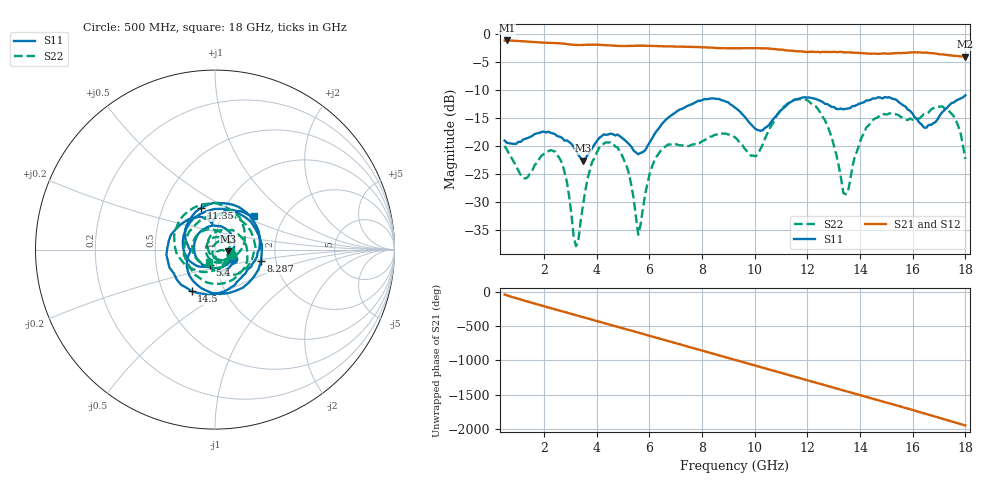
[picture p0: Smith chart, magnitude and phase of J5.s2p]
!Agilent Technologies,N5230A,MY45001360,A.07.50.67
!Agilent N5230A: A.07.50.67
!Date: Tuesday, April 16, 2024 15:56:14
!Correction: S11(Full 2 Port(1,2))
!S21(Full 2 Port(1,2))
!S12(Full 2 Port(1,2))
!S22(Full 2 Port(1,2))
!S2P File: Measurements: S11, S21, S12, S22:
# Hz S  dB  R 50
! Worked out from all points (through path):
!   201 points, 500 MHz to 18 GHz, reference 50 ohm
!   highest |S21| = -1.19 dB at 587.5 MHz (marker M1); lowest = -4.1 dB at 18 GHz (marker M2)
!   group delay of S21, straight-line fit = 300 ps
!   lowest |S11| = -22.6 dB at 3.475 GHz (marker M3), VSWR 1.16, Z = 57.9 - j1.15 ohm
!   |S11| at or under -10 dB: start of sweep to end of sweep
!   |S22| runs from -37.8 to -11.6 dB; largest |S21 - S12| = 0.0072
!   S11 on the Smith chart (normalised r, x): 500 MHz: 1.21, -0.13; 5.4 GHz: 0.93, -0.16; 8.287 GHz: 1.67, -0.23; 11.35 GHz: 0.77, +0.38; 14.5 GHz: 0.70, -0.35; 18 GHz: 1.41, +0.57
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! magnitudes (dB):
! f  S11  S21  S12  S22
! 500 MHz  -19.0  -1.2  -1.2  -20.0
! 587.5 MHz  -19.4  -1.2  -1.2  -20.6
! 1.288 GHz  -18.7  -1.4  -1.4  -25.8
! 2.425 GHz  -17.9  -1.7  -1.7  -21.0
! 2.862 GHz  -19.0  -1.8  -1.8  -26.3
! 3.212 GHz  -20.8  -2.0  -2.0  -37.8
! 3.475 GHz  -22.6  -2.0  -2.0  -30.6
! 4.35 GHz  -18.0  -2.0  -2.0  -19.3
! 5.4 GHz  -20.8  -2.1  -2.1  -29.3
! 5.575 GHz  -21.5  -2.1  -2.1  -35.8
! 6.362 GHz  -16.8  -2.2  -2.2  -21.3
! 8.287 GHz  -11.6  -2.5  -2.5  -18.3
! 9.25 GHz  -13.2  -2.6  -2.6  -18.4
! 10.04 GHz  -17.0  -2.6  -2.6  -21.9
! 11.35 GHz  -12.2  -3.0  -3.0  -12.2
! 12.22 GHz  -11.5  -3.2  -3.2  -12.6
! 13.45 GHz  -13.4  -3.3  -3.3  -28.6
! 14.5 GHz  -11.5  -3.5  -3.5  -15.3
! 15.11 GHz  -11.3  -3.6  -3.5  -14.2
! 16.43 GHz  -16.7  -3.4  -3.4  -14.3
! 17.3 GHz  -13.2  -3.8  -3.8  -13.4
! 18 GHz  -11.0  -4.1  -4.1  -22.3
